FUNCTION_BLOCK FB_EtherCATFrameDiag
VAR_INPUT
	wFrmXWcState 		: WORD;				// FrmXWcState
	wReqZeroMask 		: WORD := 16#FFFF;	// mask, bit TRUE: require wFrmXWcState.bit = FALSE, bit FALSE: ignore wFrmXWcState.bit *)
END_VAR
VAR_OUTPUT
	bFrameWcStateOK		: BOOL;				// result of fram state check
END_VAR
VAR
END_VAR

(* mask out ignored error bits and compare result against 0 *)
bFrameWcStateOK := ((wFrmXWcState AND wReqZeroMask) = 0);

END_FUNCTION_BLOCK
